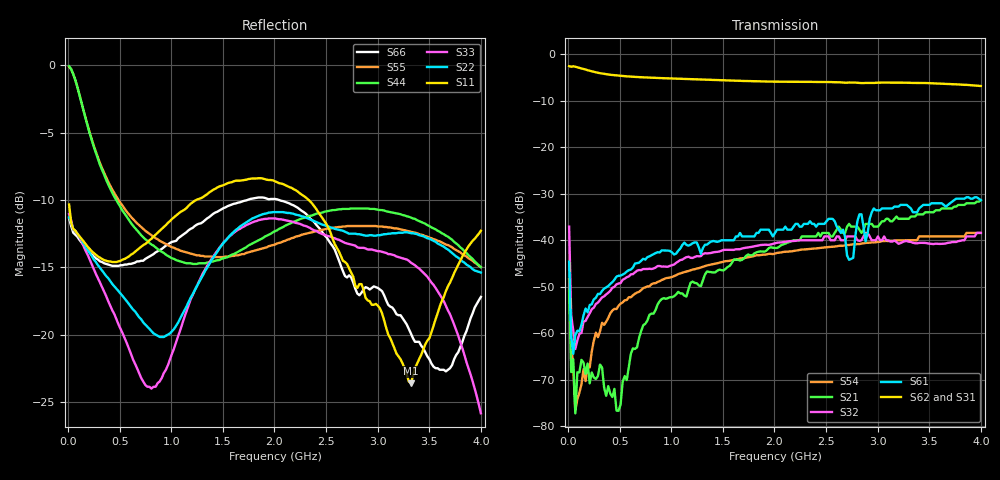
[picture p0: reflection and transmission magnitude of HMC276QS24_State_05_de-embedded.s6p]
! Hittite Microwave Corporation
! 20 Alpha Road
! Chelmsford, MA 01824
! Tel: 978-250-3343
! Fax: 978-250-3373
! Device: HMC276QS24, 0.7-3.0 GHz, GaAS MMIC 4x2 Switch Matrix in 24-lead QSOP package
! Misc: Data was de-embedded to package pins.
!  Port 1 = OP1
!  Port 2 = VL
!  Port 3 = VH
!  Port 4 = HH
!  Port 5 = HL
!  Port 6 = OP2
!  Vdd = +5 V
!  Vctl = 0 V[Logic 0] / +5 V[Logic 1]
!  State 05,  VH to OP1,  VL to OP2
!  Control Lines (Logic)
!  HV 1 = 0, Tone 1 = 1
!  HV 2 = 0, Tone 2 = 0
!  Data reformated to new Touchstone file format - Wed Jan 10 14:36:49 2007
# MHz S DB R 50
! 6 Port Network Data
! freq  dbS11  angS11  dbS12  angS12  dbS13  angS13  dbS14  angS14
!  dbS15  angS15  dbS16  angS16
!  dbS21  angS21  dbS22  angS22
!  dbS23  angS23  dbS24  angS24  dbS25  angS25  dbS26  angS26
!  dbS31  angS31  dbS32  angS32  dbS33  angS33  dbS34  angS34
!  dbS35  angS35  dbS36  angS36
!  dbS41  angS41  dbS42  angS42
!  dbS43  angS43  dbS44  angS44  dbS45  angS45  dbS46  angS46
!  dbS51  angS51  dbS52  angS52  dbS53  angS53  dbS54  angS54
!  dbS55  angS55  dbS56  angS56
!  dbS61  angS61  dbS62  angS62
!  dbS63  angS63  dbS64  angS64  dbS65  angS65  dbS66  angS66
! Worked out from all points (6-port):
!   201 points, 10 MHz to 4 GHz, reference 50 ohm
!   strongest paths, dB at 10 MHz, 1.008 GHz, 2.005 GHz, 3.002 GHz, 4 GHz:
!     S62: -2.6, -5.2, -5.9, -6.1, -6.8
!     S31: -2.8, -5.4, -6.1, -6.1, -7.0
!     S61: -44.6, -42.6, -38.4, -33.6, -31.4
!     S32: -37.1, -45.4, -40.7, -39.2, -38.4
!     S21: -50.8, -52.3, -41.7, -37.1, -31.4
!     S54: -48.3, -47.9, -42.9, -40.4, -38.4
!   lowest |S11| = -23.6 dB at 3.322 GHz (marker M1), VSWR 1.14, Z = 56.3 + j3.15 ohm
!   |S11| at or under -10 dB: start of sweep to 1.242 GHz; 2.331 GHz to end of sweep
